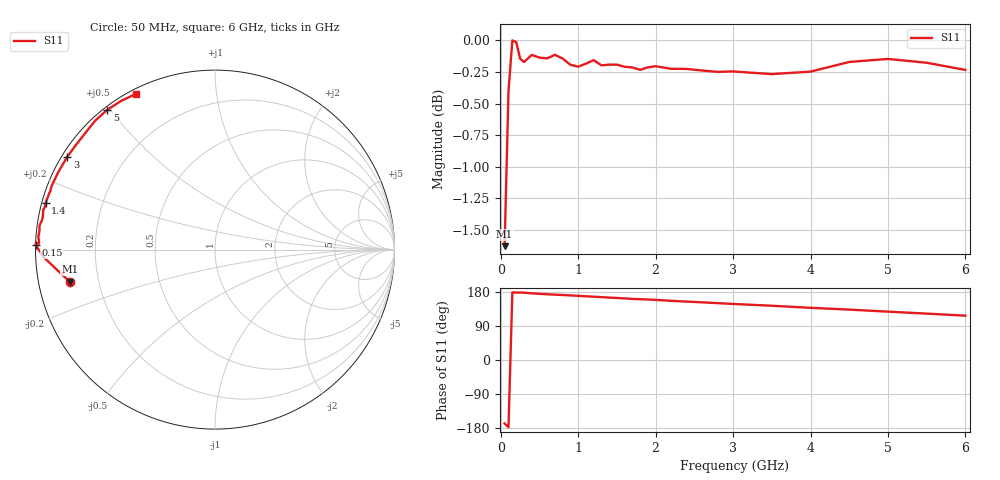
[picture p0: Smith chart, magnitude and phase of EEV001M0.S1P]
! Infineon Technologies  Discrete & RF Semiconductors
! BBY55-02W
! Si Tuning Diode in SCD-80
! VR =
! S-Parameters:  June  2000
# GHz  S  MA  R  50
!  f  S11
! GHz  MAG  ANG
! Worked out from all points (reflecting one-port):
!   34 points, 50 MHz to 6 GHz, reference 50 ohm
!   lowest |S11| = -1.6 dB at 50 MHz (marker M1), VSWR 10.70, Z = 4.73 - j5.43 ohm
!   phase of S11 starts at -168 deg and turns -76 deg over the sweep
!   S11 on the Smith chart (normalised r, x): 50 MHz: 0.09, -0.11; 150 MHz: 0.00, +0.01; 1.4 GHz: 0.01, +0.13; 3 GHz: 0.02, +0.29; 5 GHz: 0.01, +0.49; 6 GHz: 0.02, +0.61
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0.05  0.829 -167.5
0.1  0.9546 -177.4
0.15  0.9999 178.5
0.2  0.9984 177.8
0.25  0.9835 178.1
0.3  0.9804 177.6
0.4  0.9868 175.9
0.5  0.9844 174.6
0.7  0.9869 172.4
0.8  0.9835 171.5
1  0.9763 169.3
1.2  0.9821 167.0
1.3  0.9775 165.9
1.4  0.9781 164.7
1.6  0.9762 162.5
1.7  0.9756 161.2
1.9  0.9757 159.7
2  0.9767 158.6
2.2  0.9744 156.2
2.4  0.9743 154.1
2.6  0.9729 152.2
3  0.9721 147.9
3.5  0.9697 143.2
4  0.9719 137.7
4.5  0.9805 133.0
5  0.9832 127.6
5.5  0.9798 122.4
6  0.9734 117.0
